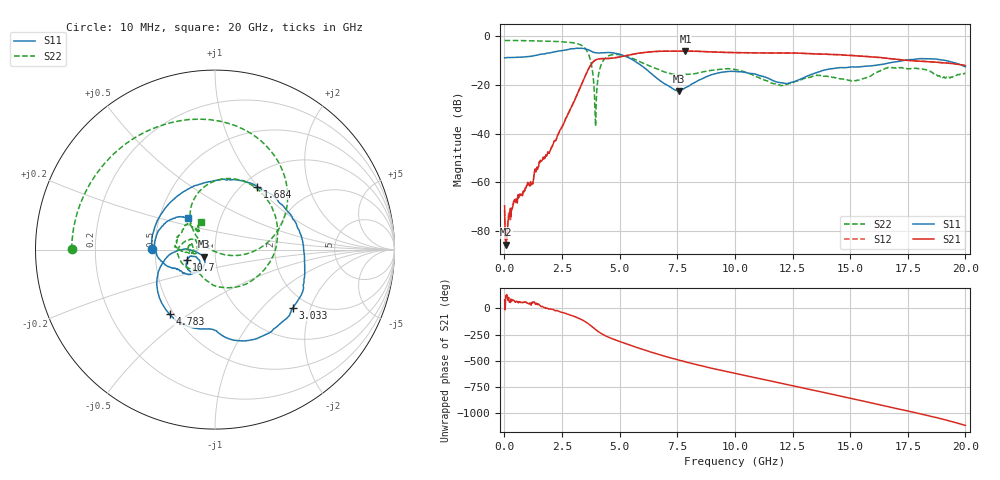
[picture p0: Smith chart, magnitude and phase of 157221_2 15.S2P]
!  2-Port S-parameters saved by WinCal
! VAR MeasName=S-Parameters (CALIBRATED_DATA) read from VNA (N5242A)
! VAR MeasDate=2015-5-26 16:48:07
! VAR NAME=157221_2 15
! VAR FILENAME=157221_2 15.S2P
! VAR DATE=2015-5-26 16:48:07
! VAR PHYS_PORTS=1,2
# Hz S DB R 50
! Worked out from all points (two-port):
!   801 points, 10 MHz to 20 GHz, reference 50 ohm
!   highest |S21| = -6.28 dB at 7.856 GHz (marker M1); lowest = -85.3 dB at 84.96 MHz (marker M2)
!   |S21| within 3 dB of the highest: 4.611 GHz to 16.63 GHz (12.02 GHz wide, 113 % of centre)
!   lowest |S11| = -22.6 dB at 7.556 GHz (marker M3), VSWR 1.16, Z = 44 - j3.54 ohm
!   |S11| at or under -10 dB: 5.589 GHz to 17.44 GHz (11.85 GHz wide, 103 % of centre); 19.05 GHz to end of sweep
!   |S22| runs from -37.0 to -2.0 dB; largest |S21 - S12| = 0.0087
!   S11 on the Smith chart (normalised r, x): 10 MHz: 0.48, +0.00; 1.684 GHz: 1.16, +0.99; 3.033 GHz: 1.67, -1.53; 4.783 GHz: 0.47, -0.42; 10.7 GHz: 0.72, -0.09; 20 GHz: 0.70, +0.26
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1e7  -9.08 179.4  -69.55 81.8  -71.41 140.8  -1.96 179.8
8.49625e7  -9.00 174.0  -85.35 125.8  -81.46 91.2  -1.96 177.9
1.684162e9  -7.49 56.2  -49.81 13.3  -49.67 13.2  -2.19 137.5
3.033488e9  -5.31 -36.6  -26.69 -76.8  -26.64 -76.8  -2.99 84.6
3.358325e9  -5.18 -59.2  -19.65 -107.4  -19.59 -107.6  -4.03 59.9
3.70815e9  -6.09 -82.5  -12.61 -157.6  -12.58 -157.9  -9.17 14.4
3.958025e9  -7.00 -91.0  -9.93 157.1  -9.91 157.0  -37.01 -157.1
4.232888e9  -6.98 -99.2  -9.40 115.7  -9.36 115.5  -11.11 118.2
4.782612e9  -7.13 -125.1  -9.08 61.0  -9.04 60.6  -7.67 65.9
5.732138e9  -10.85 -168.3  -7.31 -12.9  -7.30 -13.4  -9.99 -10.9
6.681662e9  -17.87 -177.3  -6.39 -80.2  -6.39 -80.4  -13.74 -87.7
7.556225e9  -22.58 -147.4  -6.31 -134.1  -6.31 -134.5  -15.92 -126.3
7.856075e9  -21.22 -129.8  -6.28 -151.5  -6.28 -151.8  -15.82 -134.7
8.755625e9  -16.78 -125.1  -6.55 159.1  -6.53 158.8  -14.56 -149.0
1.0005e10  -14.60 -146.2  -6.92 97.6  -6.91 97.1  -13.83 177.8
1.070465e10  -15.42 -159.4  -7.02 64.5  -7.03 64.2  -15.75 161.6
1.205398e10  -19.32 -151.4  -7.05 1.1  -7.05 0.7  -20.35 -179.2
1.335332e10  -15.69 -130.2  -7.41 -61.3  -7.36 -61.5  -16.68 -179.2
1.525238e10  -12.82 -149.6  -8.25 -152.7  -8.14 -153.2  -18.45 -177.6
1.667666e10  -11.18 -160.0  -9.33 136.8  -9.35 136.7  -13.05 176.1
1.877561e10  -9.63 160.4  -10.86 31.9  -10.88 31.7  -16.19 133.6
2e10  -12.73 131.2  -12.22 -41.2  -12.24 -42.2  -15.38 116.6
